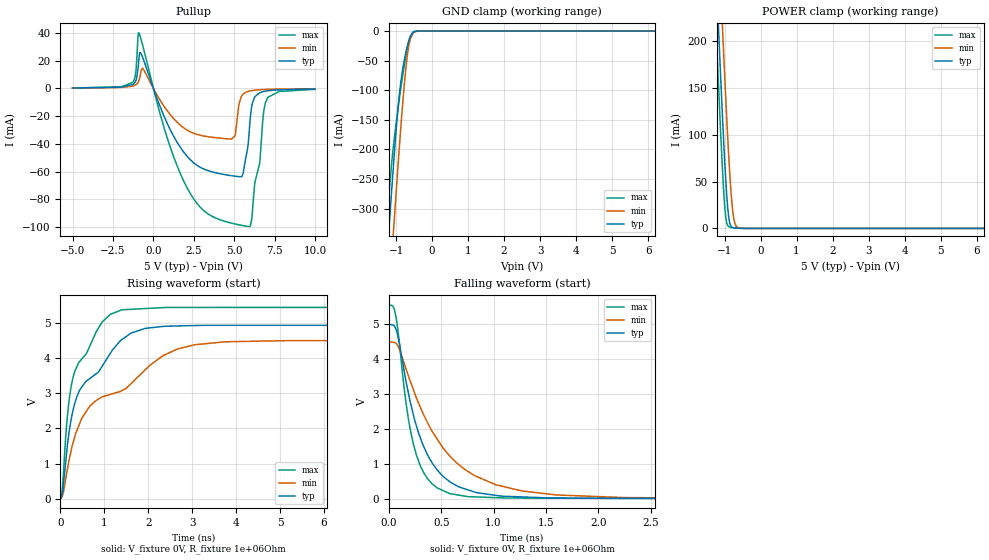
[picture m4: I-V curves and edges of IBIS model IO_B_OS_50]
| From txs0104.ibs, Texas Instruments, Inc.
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[Model]   IO_B_OS_50
Model_type   I/O_open_source
Polarity   Non-Inverting
Vinl=1.35
Vinh=3.85
Vmeas = 2.5
Vref = 0
Cref = 15pF
Rref = 1000000
|   typ   min   max
C_comp   11.90pF   11.90pF   11.90pF
[Voltage Range]   5   4.5   5.5
[Temperature Range]   27   125   -40
[Pullup Reference]   5   4.5   5.5
[Pulldown Reference]   0   0   0
[Power Clamp Reference]   5   4.5   5.5
[GND Clamp Reference]   0   0   0
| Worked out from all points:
|   slope of the pullup table from 0 to 0.75 V, typ, clamps not added: 33.4 ohm
|   GND clamp passes 1 mA (typ) near -0.49 V on its own axis
|   POWER clamp passes 1 mA (typ) near -0.77 V on its own axis
|   falling waveform, V_fixture 0V, R_fixture 1e+06Ohm: 20-80 % time 292ps typ, 522ps min, 178ps max; typ from 5 V to 0 V
|   rising waveform, V_fixture 0V, R_fixture 1e+06Ohm: 20-80 % time 951ps typ, 1.71ns min, 603ps max; typ from 0 V to 5 V
[GND Clamp]
|   Voltage   I(typ)   I(min)   I(max)
-5V       -4.062A    -4.176A    -3.992A
-1.385V   -507.7mA   -628.2mA   -437.5mA
-1.25V    -382.6mA   -501.4mA   -318.9mA
-1.175V   -315mA     -431.9mA   -259.6mA
-1.085V   -236.8mA   -349.8mA   -200.5mA
-1.04V    -199.7mA   -309.4mA   -176.1mA
-905mV    -105.2mA   -192.6mA   -112.5mA
-830mV    -69.64mA   -132.5mA   -80.43mA
-725mV    -35.06mA   -60.61mA   -40.66mA
-620mV    -11.7mA    -17.01mA   -11.93mA
-500mV    -1.186mA   -2.222mA   -728.6uA
9.985V    0A         0A         0A
[Pullup]
|   Voltage   I(typ)   I(min)   I(max)
-5V       221.6uA    177.8uA    258.3uA
-1.25V    2.85mA     1.654mA    4.455mA
-890mV    21.84mA    5.882mA    40mA
-650mV    21.88mA    14.29mA    30.51mA
850mV     -25.1mA    -16.08mA   -35.5mA
2.185V    -50.29mA   -30.78mA   -73.84mA
4.84V     -63.03mA   -36.59mA   -97.29mA
5.44V     -63.72mA   -6.026mA   -98.8mA
5.905V    -35.09mA   -2.087mA   -99.74mA
6.25V     -6.681mA   -1.378mA   -71.1mA
7.06V     -1.777mA   -759.7uA   -6.935mA
9.985V    -468uA     -287.1uA   -716uA
[POWER Clamp]
|   Voltage   I(typ)   I(min)   I(max)
-5V       3.97A      4.055A     3.919A
-1.25V    288.6mA    386.5mA    227.7mA
-1.175V   220.8mA    318.3mA    160.2mA
-1.07V    130.2mA    225.5mA    72.49mA
-1.04V    105.9mA    199.8mA    50.62mA
-965mV    51.19mA    138mA      11.75mA
-905mV    19.35mA    92.44mA    2.701mA
-860mV    6.724mA    61.93mA    1.516mA
-800mV    1.573mA    29.27mA    962.7uA
-755mV    765.5uA    13.31mA    677.5uA
-620mV    164.6uA    658.2uA    127.3uA
9.985V    0A         0A         0A
[Ramp]
R_load = 1e+06
|   typ   min   max
dV/dt_r   2.99991/9.52215e-10   2.69562/1.71027e-09   3.29993/6.06093e-10
dV/dt_f   2.99991/2.924e-10   2.69988/5.20969e-10   3.3268/1.7716e-10
[Falling Waveform]
V_fixture = 0V
V_fixture_min = 0V
V_fixture_max = 0V
R_fixture = 1e+06Ohm
C_fixture = 0F
|   Time   V(typ)   V(min)   V(max)
0s        5V         4.5V       5.552V
66.63ps   4.858V     4.452V     5.231V
184.7ps   3.05V      3.535V     2.32V
234.8ps   2.392V     3.116V     1.558V
294.9ps   1.789V     2.662V     983.5mV
471.8ps   785mV      1.66V      294.1mV
750.3ps   258.3mV    789.8mV    60.69mV
1.272ns   50.52mV    221.2mV    18.39mV
2.25ns    9.786mV    31.44mV    8.968mV
19.9ns    0V         0V         7.703mV
[Rising Waveform]
V_fixture = 0V
V_fixture_min = 0V
V_fixture_max = 0V
R_fixture = 1e+06Ohm
C_fixture = 0F
|   Time   V(typ)   V(min)   V(max)
0s        0V         7.097mV    0V
45.85ps   180.5mV    90.78mV    324.5mV
182.7ps   1.756V     1.004V     2.652V
322.5ps   2.698V     1.75V      3.609V
677.7ps   3.427V     2.644V     4.367V
949.3ps   3.768V     2.895V     5.026V
1.396ns   4.525V     3.073V     5.371V
2.344ns   4.9V       4.075V     5.436V
3.755ns   4.931V     4.463V     5.44V
19.9ns    5V         4.5V       5.5V
